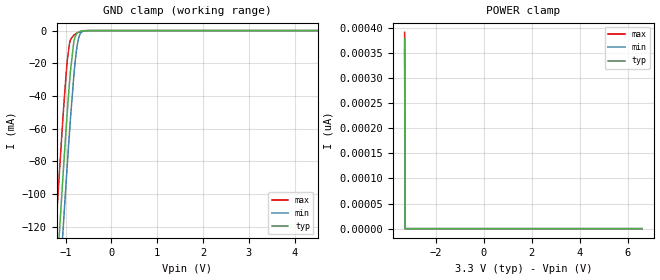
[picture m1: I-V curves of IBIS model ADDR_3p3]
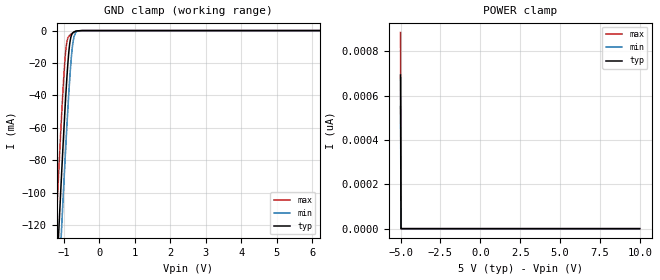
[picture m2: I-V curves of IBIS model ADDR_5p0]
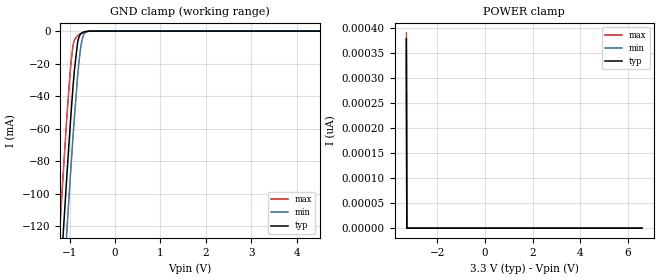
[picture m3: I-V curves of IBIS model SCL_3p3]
|Texas Instruments Incorporated
|INA220 - High or Low Side, Bi-directional CURRENT/POWER MONITOR with Two-wire
|   Interface
| Marketing part#   Digital Voltage Range   Package-type   #pins
|INA220AIDGSR   3V to 5.5V   MSOP   10
|INA220AIDGST   3V to 5.5V   MSOP   10
[IBIS Ver]   4.1
[File name]   ina220.ibs
[File Rev]   2.0
[Date]   02/03/2014
[Source]   Texas Instruments Incorporated.
   Analog-eLab, HPA
   12500 TI Blvd
   Dallas, TX -75243
   For Support e-mail: elab_ibis@list.ti.com
[Notes]   Revision History:
   2.0: 02/03/2014
   - All models have been updated with exception of package models.
   - The models with trailing _3p3 contains model for 3.3V operation.
   - The models with trailing _5p0 contains model for 5.0V operation.
   - SDA model is furter catagorized into xxxx_hs and xxxx_ls.
   xxxx_hs is for higher speed operation
   xxxx_ls is for normal and fast speed operation
   1.0: 03/29/2010
   - Initial version of the model
   - Initial Model generated from simulations in TISPICED
   - Model names with a trailing _3 contains the model for
   3.3V (3.0V and 3.6V). Model names with trailing _5 contains
   the model for 5V (4.5V and 5.5V) operation.
   - Model not matched to measurements
   - Ignore warnings related to min and max values of ccomp,
   The device process of these products is CMOS. The ccomp
   values are based on PVT variations as seen in simulations
   - C_comp: Ignore warnings related to typical values not being
   in between the minimum and maximum values for SDA_3. The c_comp
   values are  a mathematical average between the buffer's ON
   state and OFF state.
[Disclaimer]
 This product is designed as an aid for customers of Texas Instruments.
 No warranties, either expressed or implied, with respect to this third
 party software (if any) or with respect to its fitness for any
 particular purpose is claimed by Texas Instruments or the author. The
 software (if any) is provided solely on an "as is" basis. The entire
 risk as to its quality and performance is with the customer
[Copyright] (C) Copyright 2009 Texas Instruments Incorporated.
   All rights reserved.
|   INA220 - MSOP package
[Component]   INA220dgs
[Manufacturer] TI
[Package]   | MSOP
| variable   typ   min   max
R_pkg  0.055056   0.001230   0.067600
L_pkg  1.504428nH  0.574560nH  1.733960nH
C_pkg  0.291025pF  0.237080pF  0.318270pF
[Pin] signal_name  model_name  R_pin  L_pin C_pin
1   A1   ADDR   0.05947  1.58804nH  0.27948pF
2   A0   ADDR   0.05990  1.58006nH  0.30862pF
3   NC   NC   0.00123  0.57456nH  0.23708pF
4   SDA   SDA   0.05947  1.57624nH  0.30472pF
5   SCL   SCL   0.05947  1.58873nH  0.27776pF
6   VS   POWER   0.05992  1.58832nH  0.28004pF
7   GND   GND   0.06058  1.58526nH  0.30959pF
8   VBUS   TERM   0.06760  1.73396nH  0.31827pF
9   VINM   TERM   0.06191  1.61759nH  0.31358pF
10   VINP   TERM   0.06101  1.61152nH  0.28111pF
|   Model Selectors
[Model Selector]  ADDR
ADDR_3p3   3.3V digital input
ADDR_5p0   5V digital input
[Model Selector]  SCL
SCL_3p3  3.3V digital Input
SCL_5p0  5V digital Input
[Model Selector]  SDA
SDA_3p3_hs  3.3V digital I/O_open_drain, high speed
SDA_3p3_ls  3.3V digital I/O_open_drain, low/fast speed
SDA_5p0_hs  5.0V digital I/O_open_drain, high speed
SDA_5p0_ls  5.0V digital I/O_open_drain, low/fast speed
|   TERM Model
[Model] TERM
Model_type Terminator
C_comp   0   0   0
| variable   typ   min   max
[Voltage Range]   3.3V   3.0V   5.5V
[POWER Clamp Reference]  3.3V   3.0V   5.5V
[GND Clamp Reference]   0.0V   0.0V   0.0V
|Operating Temperature
[Temperature Range]   27   85   -40
| Models and submodels in the file (9): TERM (Terminator), ADDR_3p3 (Input), ADDR_5p0 (Input), SCL_3p3 (Input), SCL_5p0 (Input), SDA_3p3_hs (I/O_open_drain), SDA_3p3_ls (I/O_open_drain), SDA_5p0_hs (I/O_open_drain), SDA_5p0_ls (I/O_open_drain)
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|   Model
[Model]   ADDR_3p3
Model_type   Input
Vinl = 0.99
Vinh = 2.31
|   typ   min   max
C_comp   1.2444380e-12 1.0924310e-12 1.4001300e-12
[Voltage Range]   3.3   3   3.6
[Temperature Range]   27   85   -40
[Power Clamp Reference]   3.3   3   3.6
[GND Clamp Reference]   -0   -0   -0
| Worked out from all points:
|   GND clamp passes 1 mA (typ) near -0.72 V on its own axis
[GND Clamp]
|   Voltage   I(typ)   I(min)   I(max)
-3.3V     -1.176A    -1.208A    -1.142A
-1.231V   -166.6mA   -201mA     -129.3mA
-1.211V   -157.5mA   -191.8mA   -120.2mA
-1.132V   -121.3mA   -155.5mA   -84.37mA
-1.063V   -90.56mA   -124.3mA   -54.49mA
-983.4mV  -57.14mA   -89.81mA   -24.32mA
-924mV    -34.4mA    -65.14mA   -9.106mA
-825mV    -7.537mA   -28.64mA   -2.829mA
-765.6mV  -2.185mA   -12.41mA   -1.749mA
-706.2mV  -802.9uA   -3.59mA    -925.2uA
-518.1mV  -15.73uA   -33.56uA   -21.13uA
6.59V     0A         0A         0A
[POWER Clamp]
|   Voltage   I(typ)   I(min)   I(max)
-3.3V     379.2pA    355.3pA    391.1pA
-3.28V    0A         0A         0A
-3.27V    0A         0A         0A
6.59V     0A         0A         0A
|   Model
[Model]   ADDR_5p0
Model_type   Input
Vinl = 1.5
Vinh = 3.5
|   typ   min   max
C_comp   1.1477420e-12 1.0165180e-12 1.2888870e-12
[Voltage Range]   5   4.5   5.5
[Temperature Range]   27   85   -40
[Power Clamp Reference]   5   4.5   5.5
[GND Clamp Reference]   -0   -0   -0
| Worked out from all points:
|   GND clamp passes 1 mA (typ) near -0.72 V on its own axis
[GND Clamp]
|   Voltage   I(typ)   I(min)   I(max)
-5V       -2.019A    -2.05A     -1.986A
-1.25V    -175.5mA   -209.9mA   -138.2mA
-1.145V   -127.2mA   -161.5mA   -90.2mA
-1.13V    -120.5mA   -154.6mA   -83.53mA
-1.07V    -93.79mA   -127.6mA   -57.58mA
-1.055V   -87.25mA   -121mA     -51.35mA
-950mV    -44mA      -75.77mA   -14.53mA
-860mV    -14.64mA   -40.6mA    -3.754mA
-815mV    -6.104mA   -25.5mA    -2.622mA
-755mV    -1.796mA   -10.25mA   -1.584mA
-665mV    -405.7uA   -1.312mA   -516.6uA
9.985V    0A         0A         0A
[POWER Clamp]
|   Voltage   I(typ)   I(min)   I(max)
-5V       693.1pA    550.8pA    885.1pA
-4.97V    0A         0A         0A
-4.955V   0A         0A         0A
9.985V    0A         0A         0A
|   Model
[Model]   SCL_3p3
Model_type   Input
Vinl = 0.99
Vinh = 2.31
|   typ   min   max
C_comp   1.2013160e-12 1.0540620e-12 1.3304240e-12
[Voltage Range]   3.3   3   3.6
[Temperature Range]   27   85   -40
[Power Clamp Reference]   3.3   3   3.6
[GND Clamp Reference]   -0   -0   -0
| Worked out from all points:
|   GND clamp passes 1 mA (typ) near -0.72 V on its own axis
[GND Clamp]
|   Voltage   I(typ)   I(min)   I(max)
-3.3V     -1.176A    -1.208A    -1.142A
-1.231V   -166.6mA   -201mA     -129.3mA
-1.211V   -157.5mA   -191.8mA   -120.2mA
-1.132V   -121.3mA   -155.5mA   -84.37mA
-1.063V   -90.56mA   -124.3mA   -54.49mA
-983.4mV  -57.14mA   -89.81mA   -24.32mA
-924mV    -34.4mA    -65.14mA   -9.106mA
-825mV    -7.537mA   -28.64mA   -2.829mA
-765.6mV  -2.185mA   -12.41mA   -1.749mA
-706.2mV  -802.9uA   -3.59mA    -925.2uA
-518.1mV  -15.73uA   -33.56uA   -21.13uA
6.59V     0A         0A         0A
[POWER Clamp]
|   Voltage   I(typ)   I(min)   I(max)
-3.3V     379.2pA    355.3pA    391.1pA
-3.28V    0A         0A         0A
-3.27V    0A         0A         0A
6.59V     0A         0A         0A
